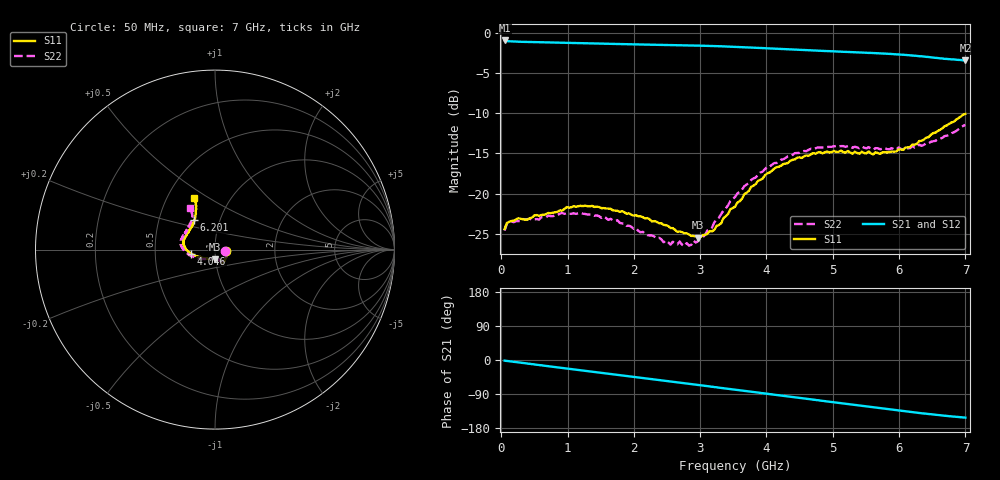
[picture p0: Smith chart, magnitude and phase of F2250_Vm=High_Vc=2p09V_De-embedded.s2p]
! Integrated Device Technology
! Corporate Headquarters
! 6024 Silver Creek Valley Road
! San Jose, CA 95138  USA
! Phone:  1-408-284-8200
! Toll Free:  1-800-223-1366
! Webpage:  http://www.idt.com/
! Timing and RF Division
! 515 Groton Road, Suite 102
! Westford, MA 01886-6024
! Device:  F2250
! Description: Voltage Variable RF Attenuator
! Frequency:  50.0 -  6000.00 MHz
! Package:  3x3 mm Thin QFN Plastic Package: 16 pin
! Ports:  2 RF, 3 DC
!  Pin  1  = GND
!  Pin  2  = NC
!  Pin  3  = RF1  = Port 1
!  Pin  4  = NC
!  Pin  5  = GND
!  Pin  6  = GND
!  Pin  7  = GND
!  Pin  8  = GND
!  Pin  9  = NC
!  Pin 10  = RF2  = Port 2
!  Pin 11  = NC
!  Pin 12  = GND
!  Pin 13  = GND
!  Pin 14  = VCNTRL
!  Pin 15  = VDD
!  Pin 16  = VMODE
! Vcntrl:  2.090 Volts
! Vmode:  +3.300 Volts
! Vdd:  +3.30  Volts
! Current:  1.318 mA
! Data:  The device was measured on a the F2250 evaluation board which has
!  individual transmission lines to the RF pins.  Data was collected
!  using a calibrated network analyzer.  The evaluation board was
!  de-embedded using a TRL calibration technique.
!  The reference plane is the edge of the package pin.
! Misc:  SN 10
!  Action Tracker AT0258
! Date Measured:  2014-11-26
! Date:  2015-10-15  MJV
! Note:
!  Integrated Device Technology supplies this data as a sample of measured
!  data at the package pin for this product.  Your particular data for this
!  product may vary.
!  Data was taken at 25 degrees C.
!  Integrated Device Technology reserves the right to change this data at anytime.
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# GHz S dB R 50
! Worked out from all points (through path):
!   201 points, 50 MHz to 7 GHz, reference 50 ohm
!   highest |S21| = -0.97 dB at 50 MHz (marker M1); lowest = -3.4 dB at 7 GHz (marker M2)
!   group delay of S21, straight-line fit = 61.1 ps
!   lowest |S11| = -25.5 dB at 2.969 GHz (marker M3), VSWR 1.11, Z = 49.7 - j5.31 ohm
!   |S11| at or under -10 dB: start of sweep to end of sweep
!   |S22| runs from -26.5 to -11.5 dB; largest |S21 - S12| = 0.0019
!   S11 on the Smith chart (normalised r, x): 50 MHz: 1.13, -0.02; 4.046 GHz: 0.76, -0.03; 6.201 GHz: 0.75, +0.26; 7 GHz: 0.68, +0.44
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0.05  -24.41 -9.3  -0.97 -1.8  -0.97 -1.8  -24.61 -9.8
0.08475  -23.63 -8.5  -1.04 -2.5  -1.04 -2.5  -23.71 -8.8
0.1195  -23.52 -9.1  -1.07 -3.3  -1.07 -3.2  -23.52 -8.3
0.91875  -22.12 -46.2  -1.26 -21.0  -1.26 -21.1  -22.40 -48.7
1.2315  -21.56 -54.0  -1.33 -27.9  -1.33 -27.9  -22.51 -59.1
1.75275  -22.14 -60.9  -1.42 -39.1  -1.42 -39.1  -23.31 -66.5
2.37825  -23.68 -61.2  -1.51 -52.8  -1.51 -52.8  -25.49 -68.8
2.552  -24.28 -65.5  -1.53 -56.6  -1.53 -56.6  -26.35 -75.4
2.691  -24.70 -72.7  -1.56 -59.7  -1.56 -59.7  -25.96 -82.5
2.7605  -24.94 -74.6  -1.57 -61.3  -1.57 -61.3  -26.54 -86.8
2.969  -25.46 -90.5  -1.61 -65.9  -1.61 -66.0  -25.92 -104.5
3.21225  -24.51 -119.8  -1.66 -71.4  -1.66 -71.5  -23.58 -128.3
3.525  -21.63 -146.8  -1.76 -78.5  -1.76 -78.5  -20.43 -146.9
3.76825  -19.16 -160.5  -1.85 -84.0  -1.85 -84.0  -18.31 -158.2
4.04625  -17.38 -170.7  -1.96 -90.2  -1.96 -90.2  -16.65 -168.7
4.4285  -15.75 178.7  -2.11 -98.6  -2.12 -98.6  -14.97 179.7
4.7065  -14.98 171.5  -2.21 -104.8  -2.21 -104.8  -14.48 173.8
5.054  -14.83 163.3  -2.34 -112.4  -2.34 -112.5  -14.09 166.6
5.85325  -14.86 137.1  -2.64 -129.9  -2.64 -130.1  -14.49 147.7
6.20075  -13.90 125.2  -2.85 -137.7  -2.85 -137.7  -14.10 138.6
6.54825  -12.43 116.9  -3.12 -144.7  -3.12 -144.8  -13.45 127.2
7  -10.10 111.8  -3.44 -152.0  -3.45 -152.1  -11.46 120.9
